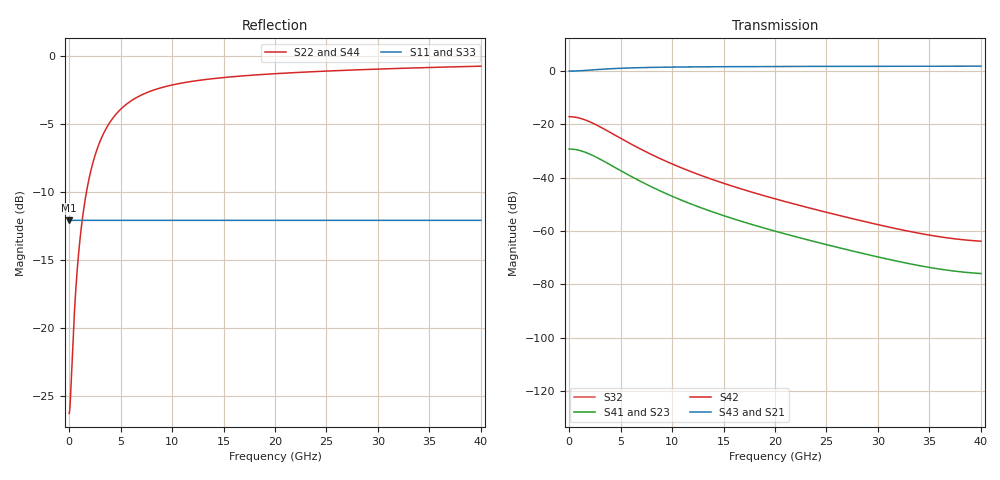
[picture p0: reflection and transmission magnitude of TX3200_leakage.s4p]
# hz S ri R 50
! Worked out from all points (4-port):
!   20000 points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, 2 MHz to 40 GHz, reference 50 ohm
!   strongest paths, dB at 2 MHz, 10 GHz, 20 GHz, 30 GHz, 40 GHz:
!     S43: -0.1, 1.4, 1.6, 1.7, 1.8
!     S21: -0.1, 1.4, 1.6, 1.7, 1.8
!     S42: -17.1, -34.8, -47.9, -57.6, -63.8
!     S41: -29.3, -47.0, -60.0, -69.7, -75.9
!     S23: -29.3, -47.0, -60.0, -69.7, -75.9
!     S32: -, -, -, -, -
!   lowest |S11| = -12.1 dB at 2 MHz (marker M1), VSWR 1.66, Z = 83 + j0 ohm
!   |S11| at or under -10 dB: start of sweep to end of sweep
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2000000  0.2482 0  0 0  0 0  0 0
         0.988 0.000109  0.0484 -0.00044  -0.0345 3.6e-05  0.1388 -0.000145
         0 0  0 0  0.2482 0  0 0
         -0.0345 3.6e-05  0.1388 -0.000145  0.9892 0.000107  0.0435 -0.000433
7.98e8  0.2482 0  0 0  0 0  0 0
        0.9962 0.0407  0.0151 -0.1641  -0.0304 0.013  0.1226 -0.0524
        0 0  0 0  0.2482 0  0 0
        -0.0304 0.013  0.1226 -0.0524  0.9972 0.0403  0.0111 -0.1624
1.69e9  0.2482 0  0 0  0 0  0 0
        1.019 0.076  -0.0785 -0.3062  -0.02 0.0214  0.0804 -0.0864
        0 0  0 0  0.2482 0  0 0
        -0.02 0.0214  0.0804 -0.0864  1.02 0.0754  -0.0808 -0.3038
5.374e9  0.2482 0  0 0  0 0  0 0
         1.12 0.1088  -0.4854 -0.4386  0.00478 0.0114  -0.0193 -0.046
         0 0  0 0  0.2482 0  0 0
         0.00478 0.0114  -0.0192 -0.046  1.121 0.1092  -0.4859 -0.4401
1.0432e10  0.2482 0  0 0  0 0  0 0
           1.175 0.0867  -0.7048 -0.3494  0.00363 0.00199  -0.0146 -0.00804
           0 0  0 0  0.2482 0  0 0
           0.00363 0.00199  -0.0146 -0.00804  1.176 0.0872  -0.7085 -0.3512
1.9382e10  0.2482 0  0 0  0 0  0 0
           1.203 0.0623  -0.8184 -0.2511  0.00108 -1.96e-05  -0.00434 7.88e-05
           0 0  0 0  0.2482 0  0 0
           0.00108 -1.88e-05  -0.00434 7.59e-05  1.204 0.062  -0.8226 -0.25
4e10  0.2482 0  0 0  0 0  0 0
      1.223 0.0423  -0.8994 -0.1703  6.54e-06 -0.000161  -2.64e-05 0.000647
      0 0  0 0  0.2482 0  0 0
      7.12e-06 -0.00016  -2.87e-05 0.000646  1.223 0.0419  -0.9006 -0.1687
